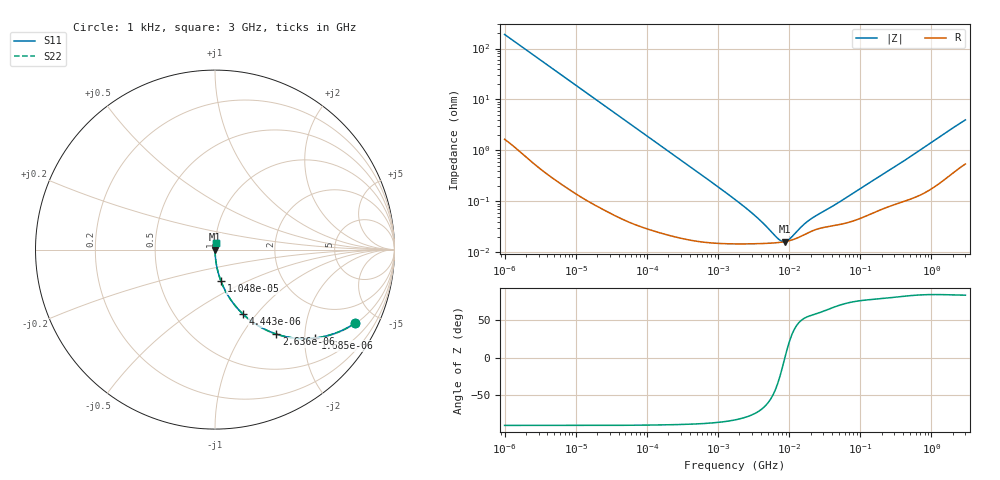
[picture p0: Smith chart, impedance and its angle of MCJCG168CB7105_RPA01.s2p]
! MCJCG168CB7105_RPA01  S-PARAMETER MODEL  ( Standard Model )
! Model Generated by TAIYO YUDEN Corporation (http://www.ty-top.com)
! Version 1.0
! TAIYO YUDEN Control No. 220601
! Copyright(c) 2015 TAIYO YUDEN CO.,LTD. All Rights Reserved.
! Product Description (link to TY-COMPAS)
! https://ds.yuden.co.jp/TYCOMPAS/or/detail?pn=MCJCG168CB7105KRPA01&u=M
! Products Name : Multilayer Ceramic Capacitors
! Characteristics :
!  Capacitance : 1 [uF] , Rated Voltage : 35 [V] , TCC : X7R
!  Case Size : 1.6 x 0.8 / 0.063 x 0.031 [mm/inch] , Thickness : 0.8 / 0.031 [mm/inch]
!  (Conditions: Temperature = 25 [degC] , DC Bias Voltage = 0 [V])
! External Node Assignments :
!  1  o---| |---o  2
! GND o---------o GND
! Frequency Range : 1kHz  -  3GHz  [ 401 STEP ]
# MHZ S RI R 50
! Freq[MHz].  S11 Real  S11 Imag  S21 Real  S21 Imag  S12 Real  S12 Imag  S22 Real  S22 Imag
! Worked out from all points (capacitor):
!   401 points, 1 kHz to 3 GHz, reference 50 ohm
!   read as one part in series: C = 841 nF near 1.077 kHz
!   lowest |Z| = 16.2 mohm at 8.607 MHz (marker M1)
!   series resonance near 8.714 MHz, so ESL is about 400 pH
!   S11 on the Smith chart (normalised r, x): 1 kHz: 1.03, -3.78; 1.685 kHz: 1.02, -2.25; 2.636 kHz: 1.01, -1.44; 4.443 kHz: 1.01, -0.86; 10.47 kHz: 1.00, -0.36; 3 GHz: 1.01, +0.08
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0.001  0.7788 -0.4107  0.2212 0.4107  0.2212 0.4107  0.7788 -0.4107
0.001251  0.6941 -0.4565  0.3059 0.4565  0.3059 0.4565  0.6941 -0.4565
0.001685  0.5577 -0.4926  0.4423 0.4926  0.4423 0.4926  0.5577 -0.4926
0.002636  0.3425 -0.4709  0.6575 0.4709  0.6575 0.4709  0.3425 -0.4709
0.004443  0.1566 -0.3599  0.8434 0.3599  0.8434 0.3599  0.1566 -0.3599
0.006451  0.0818 -0.2705  0.9182 0.2705  0.9182 0.2705  0.0818 -0.2705
0.010475  0.0334 -0.1759  0.9666 0.1759  0.9666 0.1759  0.0334 -0.1759
0.01216  0.0252 -0.1529  0.9748 0.1529  0.9748 0.1529  0.0252 -0.1529
0.033275  0.00385 -0.0574  0.9961 0.0574  0.9961 0.0574  0.00385 -0.0574
0.147855  0.000414 -0.0131  0.9996 0.0131  0.9996 0.0131  0.000414 -0.0131
1.732051  0.000147 -0.00108  0.9999 0.00108  0.9999 0.00108  0.000147 -0.00108
3.651041  0.000148 -0.00044  0.9999 0.00044  0.9999 0.00044  0.000148 -0.00044
7.143107  0.000156 -8.97e-05  0.9998 8.97e-05  0.9998 8.97e-05  0.000156 -8.97e-05
7.988506  0.000159 -3.9e-05  0.9998 3.9e-05  0.9998 3.9e-05  0.000159 -3.9e-05
8.606987  0.000162 -5.5e-06  0.9998 5.5e-06  0.9998 5.5e-06  0.000162 -5.5e-06
9.991309  0.000169 6.14e-05  0.9998 -6.14e-05  0.9998 -6.14e-05  0.000169 6.14e-05
15.62917  0.000215 0.000263  0.9998 -0.000263  0.9998 -0.000263  0.000215 0.000263
21.06097  0.000263 0.00039  0.9997 -0.00039  0.9997 -0.00039  0.000263 0.00039
47.83217  0.000345 0.000854  0.9997 -0.000854  0.9997 -0.000854  0.000345 0.000854
256.0921  0.000812 0.004  0.9992 -0.004  0.9992 -0.004  0.000812 0.004
1847.629  0.00393 0.0253  0.9961 -0.0253  0.9961 -0.0253  0.00393 0.0253
3000  0.00691 0.0389  0.9931 -0.0389  0.9931 -0.0389  0.00691 0.0389
